| IBIS File
| Lattice Semiconductor Corporation
|[Doc Num]   FPGA-MD-02094  ver. 3.0
[IBIS ver]   4.2
[File name]   ecp5u.ibs
[File Rev]   3.0
[Date]   Mon Mar 10 17:47:18 PDT 2025
[Source]   Lattice Semiconductor umc40lp Process
[Notes]   Device: LFE5U-12F   Final
   Device: LFE5U-25F   Final
   Device: LFE5U-45F   Final
   Device: LFE5U-85F   Final
   Device: LFE5UM-25F   Final
   Device: LFE5UM-45F   Final
   Device: LFE5UM-85F   Final
   Device: LFE5UM5G-25F   Final
   Device: LFE5UM5G-45F   Final
   Device: LFE5UM5G-85F   Final
   Device: LAE5U-12F   Final
   Device: LAE5UM-25F   Final
   Device: LAE5UM-45F   Final
   Device: LAE5UM-85F   Final
   Lattice Semiconductor has worked hard to ensure the
   models below are accurate and complete.  However, the
   data below was generated using simulation of the
   input/output model files for the silicon.  Therefore,
   the data below is for reference and initial design
   purposes only.
   Lattice Semiconductor grants permission to use this
   data for use in printed circuit design using this
   Lattice programmable logic device.  Other use of this
   code, including the selling or duplication of any
   portion is strictly prohibited.
|   NAMING CONVENTION
   The IBIS [Model] header is limited by the specification to a
   total of characters.  With such a set of characters available
   for naming models it becomes important to attempt to
   meaningfully encode the IO standards so they fit within the
   twenty character limit.  It would seem that twenty characters
   would provide room enough for describing IO's.  However, the
   PLD IO structure continues to grow more and more complex.  The
   complexity is making the twenty characters insuffiently
   descriptive.  In order to overcome this issue the naming
   convention described below is implemented to resolve the issue.
The twenty character space is managed as follows:
   bbbvvvsdddprttaaoixx
   b = standard
   v = voltage (x.xx V)
   s = slew code
   d = drive (xx.x ma)
   p = pullmode code
   r = impedance
   t = termination code
   o = diff resistor code
   i = diff  current code
   x = reserved
   standard
   LVCMOS   lvc
   lvcmosd   lvd
   LVDS25e   lve
   LVTTL   lvt
   lvttld   ltd
   sstl_I   ss1
   sstl_II   ss2
   sstld_I   s1d
   sstld_II   s2d
   hsul12   hs1
   hsul12d   h1d
   lvds   lvs
   blvds25   blv
   blvds25e   blv
   mlvds   mlv
   mlvds25e   mle
   lvpecl33   lvp
   lvpecl33e   lvp
   sublvds   slv
   slvs   svs
   slvs15e   sve
   mipi   mip
   vref1   vr1
   slew
   na   a
   fast   f
   slow   s
   pullmode
   off   a
   clamp   e
   impedance
   off   a
   termination
   off   aa
   50   cc
   75   dd
   150   ee
   differential resistor
   off   a
   100   b
   differential current
   NA   a
   3.5   c
   Reserved   IO type
   in   input only
   ou   output
   io   I/O
   od   Open drain
   on   Inverting differential I/O
   (signal name only)
   op   Non-Inverting differential I/O
   (signal name only)
   All the IO models are generated with pull mode set to none.
   Lattice Semiconductor Corporation
   5555 NE Moore Court
   Hillsboro, OR 97214
   U.S.A
   TEL: 1-800-Lattice (USA and Canada)
   408-826-6000 (other locations)
   web: http://www.latticesemi.com/
   email: techsupport@latticesemi.com
The IBIS models by default includes the worst case package data
under [package].  If detailed package model is required , it can be
enable using [package model] keyword.
The .pkg files are included in the zip file with the IBIS models.
The .pkg file has to be located in the same directory as IBIS file.
[Disclaimer] This IBIS source code is intended as a design reference
   which illustrates how the Lattice Semiconductor device operates.
   It is the user's responsibility to verify their design for
   consistency and functionality through the use of formal
   verification methods.  Lattice Semiconductor provides no warranty
   regarding the use or functionality of this data.
[Copyright]   Copyright 2007 by Lattice Semiconductor Corporation
|   Component SAPPHIRE
[Component]   SAPPHIRE
[Manufacturer]   Lattice Semiconductor Corp.
[Package]
|csfBGA285
| variable   typ   min   max
R_pkg   64.450m   23.9m   84m
L_pkg   1.395nH   0.37nH   2.15nH
C_pkg   0.56pF   0.19pF   0.65pF
|caBGA256
| variable   typ   min   max
|R_pkg   301.88m   168.88m   475.12m
|L_pkg   4.862nH   2.153nH   8.583nH
|C_pkg   0.654pF   0.3926pF   1.017pF
|caBGA381
| variable   typ   min   max
|R_pkg   84.450m   81.900m   87.000m
|L_pkg   5.395nH   4.379nH   6.81nH
|C_pkg   0.806pF   0.677pF   1.135pF
|caBGA554
| variable   typ   min   max
|R_pkg   740m   471.54m   505m
|L_pkg   6.1nH   4.8nH   8.1nH
|C_pkg   1.01pF   0.74pF   1.304pF
|caBGA756
| variable   typ   min   max
|R_pkg   284.450m   181.900m   387.000m
|L_pkg   6.395nH   5.379nH   8.411nH
|C_pkg   0.806pF   0.677pF   1.135pF
|caBGA225
| variable   typ   min   max
|R_pkg   219.18m   67.234m   502.9m
|L_pkg   1.301nH   0.5017nH   2.898nH
|C_pkg   0.5201pF   0.3141pF   0.812pF
|TQFP144
| variable   typ   min   max
|R_pkg   0.57206   0.48228   0.73831
|L_pkg   7.596e-9   6.661e-9   8.771e-9
|C_pkg   5.076e-13   4.246e-13   6.163e-13
[Pin]  signal_name   model_name   R_pin   L_pin   C_pin
1   blv250f160eaaaaaaaio   blv250f160eaaaaaaaio
2   blv250s160eaaaaaaaio   blv250s160eaaaaaaaio
3   hs1120f040eaaaaaaaio   hs1120f040eaaaaaaaio
4   hs1120f080eaaaaaaaio   hs1120f080eaaaaaaaio
5   hs1120s040eaaaaaaaio   hs1120s040eaaaaaaaio
6   hs1120s080eaaaaaaaio   hs1120s080eaaaaaaaio
7   lvc120f040eaaaaaaaio   lvc120f040eaaaaaaaio
8   lvc120f080eaaaaaaaio   lvc120f080eaaaaaaaio
9   lvc120s040eaaaaaaaio   lvc120s040eaaaaaaaio
10   lvc120s080eaaaaaaaio   lvc120s080eaaaaaaaio
11   lvc150f040eaaaaaaaio   lvc150f040eaaaaaaaio
12   lvc150f080eaaaaaaaio   lvc150f080eaaaaaaaio
13   lvc150f120eaaaaaaaio   lvc150f120eaaaaaaaio
14   lvc150s040eaaaaaaaio   lvc150s040eaaaaaaaio
15   lvc150s080eaaaaaaaio   lvc150s080eaaaaaaaio
16   lvc150s120eaaaaaaaio   lvc150s120eaaaaaaaio
17   lvc180f040eaaaaaaaio   lvc180f040eaaaaaaaio
18   lvc180f080eaaaaaaaio   lvc180f080eaaaaaaaio
19   lvc180f120eaaaaaaaio   lvc180f120eaaaaaaaio
20   lvc180s040eaaaaaaaio   lvc180s040eaaaaaaaio
21   lvc180s080eaaaaaaaio   lvc180s080eaaaaaaaio
22   lvc180s120eaaaaaaaio   lvc180s120eaaaaaaaio
23   lvc250f040eaaaaaaaio   lvc250f040eaaaaaaaio
24   lvc250f080eaaaaaaaio   lvc250f080eaaaaaaaio
25   lvc250f120eaaaaaaaio   lvc250f120eaaaaaaaio
26   lvc250s040eaaaaaaaio   lvc250s040eaaaaaaaio
27   lvc250s080eaaaaaaaio   lvc250s080eaaaaaaaio
28   lvc250s120eaaaaaaaio   lvc250s120eaaaaaaaio
29   lvc330f040eaaaaaaaio   lvc330f040eaaaaaaaio
30   lvc330f080eaaaaaaaio   lvc330f080eaaaaaaaio
31   lvc330f120eaaaaaaaio   lvc330f120eaaaaaaaio
32   lvc330f160eaaaaaaaio   lvc330f160eaaaaaaaio
33   lvc330s040eaaaaaaaio   lvc330s040eaaaaaaaio
34   lvc330s080eaaaaaaaio   lvc330s080eaaaaaaaio
35   lvc330s120eaaaaaaaio   lvc330s120eaaaaaaaio
36   lvc330s160eaaaaaaaio   lvc330s160eaaaaaaaio
37   mle250f160eaaaaaaaio   mle250f160eaaaaaaaio
38   mle250s160eaaaaaaaio   mle250s160eaaaaaaaio
39   ss1135f080eaaaaaaaio   ss1135f080eaaaaaaaio
40   ss1135s080eaaaaaaaio   ss1135s080eaaaaaaaio
41   ss1150f080eaaaaaaaio   ss1150f080eaaaaaaaio
42   ss1150s080eaaaaaaaio   ss1150s080eaaaaaaaio
43   ss1180f080eaaaaaaaio   ss1180f080eaaaaaaaio
44   ss1180s080eaaaaaaaio   ss1180s080eaaaaaaaio
45   ss2135f100eaaaaaaaio   ss2135f100eaaaaaaaio
46   ss2135s100eaaaaaaaio   ss2135s100eaaaaaaaio
47   ss2150f100eaaaaaaaio   ss2150f100eaaaaaaaio
48   ss2150s100eaaaaaaaio   ss2150s100eaaaaaaaio
49   ss2180f160eaaaaaaaio   ss2180f160eaaaaaaaio
50   ss2180s160eaaaaaaaio   ss2180s160eaaaaaaaio
51   h1d120f080eaaaaaaaio   h1d120f080eaaaaaaaio
52   h1d120s080eaaaaaaaio   h1d120s080eaaaaaaaio
53   h1d120f040eaaaaaaaio   h1d120f040eaaaaaaaio
54   h1d120s040eaaaaaaaio   h1d120s040eaaaaaaaio
55   lvd250f120eaaaaaaaio   lvd250f120eaaaaaaaio
56   lvd250f080eaaaaaaaio   lvd250f080eaaaaaaaio
57   lvd250s080eaaaaaaaio   lvd250s080eaaaaaaaio
58   lvd250s040eaaaaaaaio   lvd250s040eaaaaaaaio
59   lvd250s120eaaaaaaaio   lvd250s120eaaaaaaaio
60   lvd250f040eaaaaaaaio   lvd250f040eaaaaaaaio
61   lvd330f120eaaaaaaaio   lvd330f120eaaaaaaaio
62   lvd330s160eaaaaaaaio   lvd330s160eaaaaaaaio
63   lvd330s040eaaaaaaaio   lvd330s040eaaaaaaaio
64   lvd330f080eaaaaaaaio   lvd330f080eaaaaaaaio
65   lvd330s120eaaaaaaaio   lvd330s120eaaaaaaaio
66   lvd330s080eaaaaaaaio   lvd330s080eaaaaaaaio
67   lvd330f160eaaaaaaaio   lvd330f160eaaaaaaaio
68   lvd330f040eaaaaaaaio   lvd330f040eaaaaaaaio
69   ltd330f120eaaaaaaaio   ltd330f120eaaaaaaaio
70   ltd330s160eaaaaaaaio   ltd330s160eaaaaaaaio
71   ltd330s040eaaaaaaaio   ltd330s040eaaaaaaaio
72   ltd330f080eaaaaaaaio   ltd330f080eaaaaaaaio
73   ltd330s120eaaaaaaaio   ltd330s120eaaaaaaaio
74   ltd330s080eaaaaaaaio   ltd330s080eaaaaaaaio
75   ltd330f160eaaaaaaaio   ltd330f160eaaaaaaaio
76   ltd330f040eaaaaaaaio   ltd330f040eaaaaaaaio
77   lvt330f120eaaaaaaaio   lvt330f120eaaaaaaaio
78   lvt330s160eaaaaaaaio   lvt330s160eaaaaaaaio
79   lvt330s040eaaaaaaaio   lvt330s040eaaaaaaaio
80   lvt330f080eaaaaaaaio   lvt330f080eaaaaaaaio
81   lvt330s120eaaaaaaaio   lvt330s120eaaaaaaaio
82   lvt330s080eaaaaaaaio   lvt330s080eaaaaaaaio
83   lvt330f160eaaaaaaaio   lvt330f160eaaaaaaaio
84   lvt330f040eaaaaaaaio   lvt330f040eaaaaaaaio
85   s1d150s080eaaaaaaaio   s1d150s080eaaaaaaaio
86   s1d150f080eaaaaaaaio   s1d150f080eaaaaaaaio
87   s2d150f100eaaaaaaaio   s2d150f100eaaaaaaaio
88   s2d135s100eaaaaaaaio   s2d135s100eaaaaaaaio
89   s2d150s100eaaaaaaaio   s2d150s100eaaaaaaaio
90   s2d135f100eaaaaaaaio   s2d135f100eaaaaaaaio
91   s2d180f160eaaaaaaaio   s2d180f160eaaaaaaaio
92   s1d135s080eaaaaaaaio   s1d135s080eaaaaaaaio
93   s1d180f080eaaaaaaaio   s1d180f080eaaaaaaaio
94   s2d180s160eaaaaaaaio   s2d180s160eaaaaaaaio
95   s1d135f080eaaaaaaaio   s1d135f080eaaaaaaaio
96   s1d180s080eaaaaaaaio   s1d180s080eaaaaaaaio
97   lvd250f120eaaaaaaaop   lvd250f120eaaaaaaaou
98   lvd250f120eaaaaaaaon   lvd250f120eaaaaaaaou
99   lvc150s040eaaaaaaaou   lvc150s040eaaaaaaaou
100  lvc180f120eaaaaaaaou   lvc180f120eaaaaaaaou
101  ltd330s160eaaaaaaaop   ltd330s160eaaaaaaaou
102  ltd330s160eaaaaaaaon   ltd330s160eaaaaaaaou
103  ss1150f080eaaaaaaaou   ss1150f080eaaaaaaaou
104  s2d150f100eaaaaaaaop   s2d150f100eaaaaaaaou
105  s2d150f100eaaaaaaaon   s2d150f100eaaaaaaaou
106  lvd330s120eaaaaaaaop   lvd330s120eaaaaaaaou
107  lvd330s120eaaaaaaaon   lvd330s120eaaaaaaaou
108  lvc330f080eaaaaaaaou   lvc330f080eaaaaaaaou
109  lvd250f080eaaaaaaaop   lvd250f080eaaaaaaaou
110  lvd250f080eaaaaaaaon   lvd250f080eaaaaaaaou
111  lvc180s120eaaaaaaaou   lvc180s120eaaaaaaaou
112  s2d135f100eaaaaaaaop   s2d135f100eaaaaaaaou
113  s2d135f100eaaaaaaaon   s2d135f100eaaaaaaaou
114  s1d180s080eaaaaaaaop   s1d180s080eaaaaaaaou
115  s1d180s080eaaaaaaaon   s1d180s080eaaaaaaaou
116  lvc180s080eaaaaaaaou   lvc180s080eaaaaaaaou
117  lvc250f120eaaaaaaaou   lvc250f120eaaaaaaaou
118  lvd250s120eaaaaaaaop   lvd250s120eaaaaaaaou
119  lvd250s120eaaaaaaaon   lvd250s120eaaaaaaaou
120  lvc330f040eaaaaaaaou   lvc330f040eaaaaaaaou
121  lvc180f080eaaaaaaaou   lvc180f080eaaaaaaaou
122  ss1150s080eaaaaaaaou   ss1150s080eaaaaaaaou
123  lvc330f120eaaaaaaaou   lvc330f120eaaaaaaaou
124  ss2135s100eaaaaaaaou   ss2135s100eaaaaaaaou
125  lvc120s080eaaaaaaaou   lvc120s080eaaaaaaaou
126  ss2150s100eaaaaaaaou   ss2150s100eaaaaaaaou
127  ss2135f100eaaaaaaaou   ss2135f100eaaaaaaaou
128  s2d180s160eaaaaaaaop   s2d180s160eaaaaaaaou
129  s2d180s160eaaaaaaaon   s2d180s160eaaaaaaaou
130  lvc330s120eaaaaaaaou   lvc330s120eaaaaaaaou
131  h1d120s080eaaaaaaaop   h1d120s080eaaaaaaaou
132  h1d120s080eaaaaaaaon   h1d120s080eaaaaaaaou
133  ss2180f160eaaaaaaaou   ss2180f160eaaaaaaaou
134  lvc330f160eaaaaaaaou   lvc330f160eaaaaaaaou
135  lvd330f080eaaaaaaaop   lvd330f080eaaaaaaaou
136  lvd330f080eaaaaaaaon   lvd330f080eaaaaaaaou
137  s1d180f080eaaaaaaaop   s1d180f080eaaaaaaaou
138  s1d180f080eaaaaaaaon   s1d180f080eaaaaaaaou
139  lvd330s080eaaaaaaaop   lvd330s080eaaaaaaaou
140  lvd330s080eaaaaaaaon   lvd330s080eaaaaaaaou
141  mle250s160eaaaaaaaop   mle250s160eaaaaaaaou
142  mle250s160eaaaaaaaon   mle250s160eaaaaaaaou
143  lvc330s160eaaaaaaaou   lvc330s160eaaaaaaaou
144  lvc180s040eaaaaaaaou   lvc180s040eaaaaaaaou
145  lvc330s040eaaaaaaaou   lvc330s040eaaaaaaaou
146  lvc250s120eaaaaaaaou   lvc250s120eaaaaaaaou
147  lvc250f040eaaaaaaaou   lvc250f040eaaaaaaaou
148  hs1120f080eaaaaaaaou   hs1120f080eaaaaaaaou
149  h1d120f040eaaaaaaaop   h1d120f040eaaaaaaaou
150  h1d120f040eaaaaaaaon   h1d120f040eaaaaaaaou
151  ss1180f080eaaaaaaaou   ss1180f080eaaaaaaaou
152  mle250f160eaaaaaaaop   mle250f160eaaaaaaaou
153  mle250f160eaaaaaaaon   mle250f160eaaaaaaaou
154  lvd250s040eaaaaaaaop   lvd250s040eaaaaaaaou
155  lvd250s040eaaaaaaaon   lvd250s040eaaaaaaaou
156  ltd330f080eaaaaaaaop   ltd330f080eaaaaaaaou
157  ltd330f080eaaaaaaaon   ltd330f080eaaaaaaaou
158  lvd250f040eaaaaaaaop   lvd250f040eaaaaaaaou
159  lvd250f040eaaaaaaaon   lvd250f040eaaaaaaaou
160  lvc150f080eaaaaaaaou   lvc150f080eaaaaaaaou
161  lvc330s080eaaaaaaaou   lvc330s080eaaaaaaaou
162  lvc120s040eaaaaaaaou   lvc120s040eaaaaaaaou
163  s2d180f160eaaaaaaaop   s2d180f160eaaaaaaaou
164  s2d180f160eaaaaaaaon   s2d180f160eaaaaaaaou
165  ss1135f080eaaaaaaaou   ss1135f080eaaaaaaaou
166  ltd330s120eaaaaaaaop   ltd330s120eaaaaaaaou
167  ltd330s120eaaaaaaaon   ltd330s120eaaaaaaaou
168  lvc120f040eaaaaaaaou   lvc120f040eaaaaaaaou
169  lvc150s080eaaaaaaaou   lvc150s080eaaaaaaaou
170  lvc250s080eaaaaaaaou   lvc250s080eaaaaaaaou
171  s2d135s100eaaaaaaaop   s2d135s100eaaaaaaaou
172  s2d135s100eaaaaaaaon   s2d135s100eaaaaaaaou
173  ltd330f160eaaaaaaaop   ltd330f160eaaaaaaaou
174  ltd330f160eaaaaaaaon   ltd330f160eaaaaaaaou
175  lvc250s040eaaaaaaaou   lvc250s040eaaaaaaaou
176  lvd330s160eaaaaaaaop   lvd330s160eaaaaaaaou
177  lvd330s160eaaaaaaaon   lvd330s160eaaaaaaaou
178  s1d135s080eaaaaaaaop   s1d135s080eaaaaaaaou
179  s1d135s080eaaaaaaaon   s1d135s080eaaaaaaaou
180  lvc180f040eaaaaaaaou   lvc180f040eaaaaaaaou
181  lvc120f080eaaaaaaaou   lvc120f080eaaaaaaaou
182  blv250s160eaaaaaaaop   blv250s160eaaaaaaaou
183  blv250s160eaaaaaaaon   blv250s160eaaaaaaaou
184  ltd330s080eaaaaaaaop   ltd330s080eaaaaaaaou
185  ltd330s080eaaaaaaaon   ltd330s080eaaaaaaaou
186  h1d120s040eaaaaaaaop   h1d120s040eaaaaaaaou
187  h1d120s040eaaaaaaaon   h1d120s040eaaaaaaaou
188  lvd250s080eaaaaaaaop   lvd250s080eaaaaaaaou
189  lvd250s080eaaaaaaaon   lvd250s080eaaaaaaaou
190  lvd330f040eaaaaaaaop   lvd330f040eaaaaaaaou
191  lvd330f040eaaaaaaaon   lvd330f040eaaaaaaaou
192  ss1135s080eaaaaaaaou   ss1135s080eaaaaaaaou
193  ss2180s160eaaaaaaaou   ss2180s160eaaaaaaaou
194  hs1120f040eaaaaaaaou   hs1120f040eaaaaaaaou
195  hs1120s040eaaaaaaaou   hs1120s040eaaaaaaaou
196  s1d150f080eaaaaaaaop   s1d150f080eaaaaaaaou
197  s1d150f080eaaaaaaaon   s1d150f080eaaaaaaaou
198  ltd330s040eaaaaaaaop   ltd330s040eaaaaaaaou
199  ltd330s040eaaaaaaaon   ltd330s040eaaaaaaaou
200  ltd330f120eaaaaaaaop   ltd330f120eaaaaaaaou
201  ltd330f120eaaaaaaaon   ltd330f120eaaaaaaaou
202  lvc250f080eaaaaaaaou   lvc250f080eaaaaaaaou
203  s2d150s100eaaaaaaaop   s2d150s100eaaaaaaaou
204  s2d150s100eaaaaaaaon   s2d150s100eaaaaaaaou
205  ltd330f040eaaaaaaaop   ltd330f040eaaaaaaaou
206  ltd330f040eaaaaaaaon   ltd330f040eaaaaaaaou
207  s1d150s080eaaaaaaaop   s1d150s080eaaaaaaaou
208  s1d150s080eaaaaaaaon   s1d150s080eaaaaaaaou
209  blv250f160eaaaaaaaop   blv250f160eaaaaaaaou
210  blv250f160eaaaaaaaon   blv250f160eaaaaaaaou
211  lvd330f120eaaaaaaaop   lvd330f120eaaaaaaaou
212  lvd330f120eaaaaaaaon   lvd330f120eaaaaaaaou
213  h1d120f080eaaaaaaaop   h1d120f080eaaaaaaaou
214  h1d120f080eaaaaaaaon   h1d120f080eaaaaaaaou
215  lvd330s040eaaaaaaaop   lvd330s040eaaaaaaaou
216  lvd330s040eaaaaaaaon   lvd330s040eaaaaaaaou
217  lvd330f160eaaaaaaaop   lvd330f160eaaaaaaaou
218  lvd330f160eaaaaaaaon   lvd330f160eaaaaaaaou
219  ss2150f100eaaaaaaaou   ss2150f100eaaaaaaaou
220  s1d135f080eaaaaaaaop   s1d135f080eaaaaaaaou
221  s1d135f080eaaaaaaaon   s1d135f080eaaaaaaaou
222  hs1120s080eaaaaaaaou   hs1120s080eaaaaaaaou
223  lvc150f040eaaaaaaaou   lvc150f040eaaaaaaaou
224  ss1180s080eaaaaaaaou   ss1180s080eaaaaaaaou
225  ss1150s080eaccaaaaio   ss1150s080eaccaaaaio
226  ss1150f080eaccaaaaio   ss1150f080eaccaaaaio
227  ss2150f100eaccaaaaio   ss2150f100eaccaaaaio
228  ss2135s100eaccaaaaio   ss2135s100eaccaaaaio
229  ss2150s100eaccaaaaio   ss2150s100eaccaaaaio
230  ss2135f100eaccaaaaio   ss2135f100eaccaaaaio
231  ss2180f160eaccaaaaio   ss2180f160eaccaaaaio
232  ss1135s080eaccaaaaio   ss1135s080eaccaaaaio
233  ss1180f080eaccaaaaio   ss1180f080eaccaaaaio
234  ss2180s160eaccaaaaio   ss2180s160eaccaaaaio
235  ss1135f080eaccaaaaio   ss1135f080eaccaaaaio
236  ss1180s080eaccaaaaio   ss1180s080eaccaaaaio
237  ss1150s080eaddaaaaio   ss1150s080eaddaaaaio
238  ss1150f080eaddaaaaio   ss1150f080eaddaaaaio
239  ss2150f100eaddaaaaio   ss2150f100eaddaaaaio
240  ss2135s100eaddaaaaio   ss2135s100eaddaaaaio
241  ss2150s100eaddaaaaio   ss2150s100eaddaaaaio
242  ss2135f100eaddaaaaio   ss2135f100eaddaaaaio
243  ss2180f160eaddaaaaio   ss2180f160eaddaaaaio
244  ss1135s080eaddaaaaio   ss1135s080eaddaaaaio
245  ss1180f080eaddaaaaio   ss1180f080eaddaaaaio
246  ss2180s160eaddaaaaio   ss2180s160eaddaaaaio
247  ss1135f080eaddaaaaio   ss1135f080eaddaaaaio
248  ss1180s080eaddaaaaio   ss1180s080eaddaaaaio
249  ss1150s080eaeeaaaaio   ss1150s080eaeeaaaaio
250  ss1150f080eaeeaaaaio   ss1150f080eaeeaaaaio
251  ss2150f100eaeeaaaaio   ss2150f100eaeeaaaaio
252  ss2135s100eaeeaaaaio   ss2135s100eaeeaaaaio
253  ss2150s100eaeeaaaaio   ss2150s100eaeeaaaaio
254  ss2135f100eaeeaaaaio   ss2135f100eaeeaaaaio
255  ss2180f160eaeeaaaaio   ss2180f160eaeeaaaaio
256  ss1135s080eaeeaaaaio   ss1135s080eaeeaaaaio
257  ss1180f080eaeeaaaaio   ss1180f080eaeeaaaaio
258  ss2180s160eaeeaaaaio   ss2180s160eaeeaaaaio
259  ss1135f080eaeeaaaaio   ss1135f080eaeeaaaaio
260  ss1180s080eaeeaaaaio   ss1180s080eaeeaaaaio
261  s1d150s080eaaaaabaio   s1d150s080eaaaaabaio
262  s1d150f080eaaaaabaio   s1d150f080eaaaaabaio
263  s2d150f100eaaaaabaio   s2d150f100eaaaaabaio
264  s2d135s100eaaaaabaio   s2d135s100eaaaaabaio
265  s2d150s100eaaaaabaio   s2d150s100eaaaaabaio
266  s2d135f100eaaaaabaio   s2d135f100eaaaaabaio
267  s2d180f160eaaaaabaio   s2d180f160eaaaaabaio
268  s1d135s080eaaaaabaio   s1d135s080eaaaaabaio
269  s1d180f080eaaaaabaio   s1d180f080eaaaaabaio
270  s2d180s160eaaaaabaio   s2d180s160eaaaaabaio
271  s1d135f080eaaaaabaio   s1d135f080eaaaaabaio
272  lvt330s120eaaaaaaaou   lvt330s120eaaaaaaaou
273  lvt330f080eaaaaaaaou   lvt330f080eaaaaaaaou
274  lvt330s080eaaaaaaaou   lvt330s080eaaaaaaaou
275  lvt330s160eaaaaaaaou   lvt330s160eaaaaaaaou
276  lvt330s040eaaaaaaaou   lvt330s040eaaaaaaaou
277  lvt330f160eaaaaaaaou   lvt330f160eaaaaaaaou
278  lve250f080eaaaaaaaou   lve250f080eaaaaaaaou
279  s1d180s080eaaaaabaio   s1d180s080eaaaaabaio
280  lvt330f120eaaaaaaaou   lvt330f120eaaaaaaaou
281  lvt330f040eaaaaaaaou   lvt330f040eaaaaaaaou
282  lve250s080eaaaaaaaou   lve250s080eaaaaaaaou
283  lvp330s160eaaaaaaaop   lvp330s160eaaaaaaaou
284  lvp330s160eaaaaaaaon   lvp330s160eaaaaaaaou
285  lvp330f160eaaaaaaaop   lvp330f160eaaaaaaaou
286  lvp330f160eaaaaaaaon   lvp330f160eaaaaaaaou
287  lvc150s040eaaaaaaaod   lvc150s040eaaaaaaaod
288  lvc180f120eaaaaaaaod   lvc180f120eaaaaaaaod
289  lvt330s160eaaaaaaaod   lvt330s160eaaaaaaaod
290  lvc330f080eaaaaaaaod   lvc330f080eaaaaaaaod
291  lvc180s120eaaaaaaaod   lvc180s120eaaaaaaaod
292  lvc180s080eaaaaaaaod   lvc180s080eaaaaaaaod
293  lvc250f120eaaaaaaaod   lvc250f120eaaaaaaaod
294  lvt330s120eaaaaaaaod   lvt330s120eaaaaaaaod
295  lvc330f040eaaaaaaaod   lvc330f040eaaaaaaaod
296  lvc180f080eaaaaaaaod   lvc180f080eaaaaaaaod
297  lvc330f120eaaaaaaaod   lvc330f120eaaaaaaaod
298  lvc120s080eaaaaaaaod   lvc120s080eaaaaaaaod
299  lvc330s120eaaaaaaaod   lvc330s120eaaaaaaaod
300  lvc330f160eaaaaaaaod   lvc330f160eaaaaaaaod
301  lvc330s160eaaaaaaaod   lvc330s160eaaaaaaaod
302  lvc180s040eaaaaaaaod   lvc180s040eaaaaaaaod
303  lvc330s040eaaaaaaaod   lvc330s040eaaaaaaaod
304  lvc250s120eaaaaaaaod   lvc250s120eaaaaaaaod
305  lvc250f040eaaaaaaaod   lvc250f040eaaaaaaaod
306  lvc150f080eaaaaaaaod   lvc150f080eaaaaaaaod
307  lvc330s080eaaaaaaaod   lvc330s080eaaaaaaaod
308  lvc120s040eaaaaaaaod   lvc120s040eaaaaaaaod
309  lvt330f120eaaaaaaaod   lvt330f120eaaaaaaaod
310  lvc120f040eaaaaaaaod   lvc120f040eaaaaaaaod
311  lvc150s080eaaaaaaaod   lvc150s080eaaaaaaaod
312  lvc250s080eaaaaaaaod   lvc250s080eaaaaaaaod
313  lvc250s040eaaaaaaaod   lvc250s040eaaaaaaaod
314  lvt330s040eaaaaaaaod   lvt330s040eaaaaaaaod
315  lvc180f040eaaaaaaaod   lvc180f040eaaaaaaaod
316  lvt330f160eaaaaaaaod   lvt330f160eaaaaaaaod
317  lvc120f080eaaaaaaaod   lvc120f080eaaaaaaaod
318  lvt330f080eaaaaaaaod   lvt330f080eaaaaaaaod
319  lvt330s080eaaaaaaaod   lvt330s080eaaaaaaaod
320  lvc250f080eaaaaaaaod   lvc250f080eaaaaaaaod
321  lvt330f040eaaaaaaaod   lvt330f040eaaaaaaaod
322  lvc150f040eaaaaaaaod   lvc150f040eaaaaaaaod
323  lvc150s040aaaaaaaaod   lvc150s040aaaaaaaaod
324  lvc180f120aaaaaaaaod   lvc180f120aaaaaaaaod
325  lvt330s160aaaaaaaaod   lvt330s160aaaaaaaaod
326  lvc330f080aaaaaaaaod   lvc330f080aaaaaaaaod
327  lvc180s120aaaaaaaaod   lvc180s120aaaaaaaaod
328  lvc180s080aaaaaaaaod   lvc180s080aaaaaaaaod
329  lvc250f120aaaaaaaaod   lvc250f120aaaaaaaaod
330  lvt330s120aaaaaaaaod   lvt330s120aaaaaaaaod
331  lvc330f040aaaaaaaaod   lvc330f040aaaaaaaaod
332  lvc180f080aaaaaaaaod   lvc180f080aaaaaaaaod
333  lvc330f120aaaaaaaaod   lvc330f120aaaaaaaaod
334  lvc120s080aaaaaaaaod   lvc120s080aaaaaaaaod
335  lvc330s120aaaaaaaaod   lvc330s120aaaaaaaaod
336  lvc330f160aaaaaaaaod   lvc330f160aaaaaaaaod
337  lvc330s160aaaaaaaaod   lvc330s160aaaaaaaaod
338  lvc180s040aaaaaaaaod   lvc180s040aaaaaaaaod
339  lvc330s040aaaaaaaaod   lvc330s040aaaaaaaaod
340  lvc250s120aaaaaaaaod   lvc250s120aaaaaaaaod
341  lvc250f040aaaaaaaaod   lvc250f040aaaaaaaaod
342  lvc150f080aaaaaaaaod   lvc150f080aaaaaaaaod
343  lvc330s080aaaaaaaaod   lvc330s080aaaaaaaaod
344  lvc120s040aaaaaaaaod   lvc120s040aaaaaaaaod
345  lvt330f120aaaaaaaaod   lvt330f120aaaaaaaaod
346  lvc120f040aaaaaaaaod   lvc120f040aaaaaaaaod
347  lvc150s080aaaaaaaaod   lvc150s080aaaaaaaaod
348  lvc250s080aaaaaaaaod   lvc250s080aaaaaaaaod
349  lvc250s040aaaaaaaaod   lvc250s040aaaaaaaaod
350  lvt330s040aaaaaaaaod   lvt330s040aaaaaaaaod
351  lvc180f040aaaaaaaaod   lvc180f040aaaaaaaaod
352  lvt330f160aaaaaaaaod   lvt330f160aaaaaaaaod
353  lvc120f080aaaaaaaaod   lvc120f080aaaaaaaaod
354  lvt330f080aaaaaaaaod   lvt330f080aaaaaaaaod
355  lvt330s080aaaaaaaaod   lvt330s080aaaaaaaaod
356  lvc250f080aaaaaaaaod   lvc250f080aaaaaaaaod
357  lvt330f040aaaaaaaaod   lvt330f040aaaaaaaaod
358  lvc150f040aaaaaaaaod   lvc150f040aaaaaaaaod
359  lvc120f120aaaaaaaaod   lvc120f120aaaaaaaaod
360  lvc120s120aaaaaaaaod   lvc120s120aaaaaaaaod
361  lvc150f120aaaaaaaaod   lvc150f120aaaaaaaaod
362  lvc150s120aaaaaaaaod   lvc150s120aaaaaaaaod
363  lvc180f160aaaaaaaaod   lvc180f160aaaaaaaaod
364  lvc180s160aaaaaaaaod   lvc180s160aaaaaaaaod
365  lvc250f160aaaaaaaaod   lvc250f160aaaaaaaaod
366  lvc250s160aaaaaaaaod   lvc250s160aaaaaaaaod
367  lvc120f120eaaaaaaaod   lvc120f120eaaaaaaaod
368  lvc120s120eaaaaaaaod   lvc120s120eaaaaaaaod
369  lvc150f120eaaaaaaaod   lvc150f120eaaaaaaaod
370  lvc150s120eaaaaaaaod   lvc150s120eaaaaaaaod
371  lvc180f160eaaaaaaaod   lvc180f160eaaaaaaaod
372  lvc180s160eaaaaaaaod   lvc180s160eaaaaaaaod
373  lvc250f160eaaaaaaaod   lvc250f160eaaaaaaaod
374  lvc250s160eaaaaaaaod   lvc250s160eaaaaaaaod
375  lvc120f160aaaaaaaaod   lvc120f160aaaaaaaaod
376  lvc120f160eaaaaaaaod   lvc120f160eaaaaaaaod
377  lvc120s160aaaaaaaaod   lvc120s160aaaaaaaaod
378  lvc120s160eaaaaaaaod   lvc120s160eaaaaaaaod
379  lvc150f160aaaaaaaaod   lvc150f160aaaaaaaaod
380  lvc150f160eaaaaaaaod   lvc150f160eaaaaaaaod
381  lvc150s160aaaaaaaaod   lvc150s160aaaaaaaaod
382  lvc150s160eaaaaaaaod   lvc150s160eaaaaaaaod
383  lvs250axxxeaaaaaacio   lvs250axxxeaaaaaacio
384  lvs250axxxeaaaaaacop   lvs250axxxeaaaaaacou
385  lvs250axxxeaaaaaacon   lvs250axxxeaaaaaacou
386  blv250axxxeaaaaaaain   blv250axxxeaaaaaaain
387  h1d120axxxeaaaaaaain   h1d120axxxeaaaaaaain
388  hs1120axxxeaaaaaaain   hs1120axxxeaaaaaaain
389  ltd330axxxeaaaaaaain   ltd330axxxeaaaaaaain
390  lvc120axxxeaaaaaaain   lvc120axxxeaaaaaaain
391  lvc150axxxeaaaaaaain   lvc150axxxeaaaaaaain
392  lvc180axxxeaaaaaaain   lvc180axxxeaaaaaaain
393  lvc250axxxaaaaaaaain   lvc250axxxaaaaaaaain
394  lvc250axxxeaaaaaaain   lvc250axxxeaaaaaaain
395  lvc330axxxaaaaaaaain   lvc330axxxaaaaaaaain
396  lvc330axxxeaaaaaaain   lvc330axxxeaaaaaaain
397  lvd250axxxeaaaaaaain   lvd250axxxeaaaaaaain
398  lvd330axxxeaaaaaaain   lvd330axxxeaaaaaaain
399  lvp330axxxeaaaaaaain   lvp330axxxeaaaaaaain
400  lvs250axxxeaaaaaaain   lvs250axxxeaaaaaaain
401  lvt330axxxaaaaaaaain   lvt330axxxaaaaaaaain
402  lvt330axxxeaaaaaaain   lvt330axxxeaaaaaaain
403  mlv250axxxeaaaaaaain   mlv250axxxeaaaaaaain
404  s1d135axxxeaaaaaaain   s1d135axxxeaaaaaaain
405  s1d150axxxeaaaaaaain   s1d150axxxeaaaaaaain
406  s1d180axxxeaaaaaaain   s1d180axxxeaaaaaaain
407  s2d135axxxeaaaaaaain   s2d135axxxeaaaaaaain
408  s2d150axxxeaaaaaaain   s2d150axxxeaaaaaaain
409  s2d180axxxeaaaaaaain   s2d180axxxeaaaaaaain
410  slv250axxxeaaaaaaain   slv250axxxeaaaaaaain
411  ss1135axxxeaaaaaaain   ss1135axxxeaaaaaaain
412  ss1135axxxeaccaaaain   ss1135axxxeaccaaaain
413  ss1135axxxeaddaaaain   ss1135axxxeaddaaaain
414  ss1135axxxeaeeaaaain   ss1135axxxeaeeaaaain
415  ss1150axxxeaaaaaaain   ss1150axxxeaaaaaaain
416  ss1150axxxeaccaaaain   ss1150axxxeaccaaaain
417  ss1150axxxeaddaaaain   ss1150axxxeaddaaaain
418  ss1150axxxeaeeaaaain   ss1150axxxeaeeaaaain
419  ss1180axxxeaaaaaaain   ss1180axxxeaaaaaaain
420  ss1180axxxeaccaaaain   ss1180axxxeaccaaaain
421  ss1180axxxeaddaaaain   ss1180axxxeaddaaaain
422  ss1180axxxeaeeaaaain   ss1180axxxeaeeaaaain
423  ss2135axxxeaaaaaaain   ss2135axxxeaaaaaaain
424  ss2135axxxeaccaaaain   ss2135axxxeaccaaaain
425  ss2135axxxeaddaaaain   ss2135axxxeaddaaaain
426  ss2135axxxeaeeaaaain   ss2135axxxeaeeaaaain
427  ss2150axxxeaaaaaaain   ss2150axxxeaaaaaaain
428  ss2150axxxeaccaaaain   ss2150axxxeaccaaaain
429  ss2150axxxeaddaaaain   ss2150axxxeaddaaaain
430  ss2150axxxeaeeaaaain   ss2150axxxeaeeaaaain
431  ss2180axxxeaaaaaaain   ss2180axxxeaaaaaaain
432  ss2180axxxeaccaaaain   ss2180axxxeaccaaaain
433  ss2180axxxeaddaaaain   ss2180axxxeaddaaaain
434  ss2180axxxeaeeaaaain   ss2180axxxeaeeaaaain
435  svs120axxxeaaaaaaain   svs120axxxeaaaaaaain
436  s2d180axxxeaaaaabain   s2d180axxxeaaaaabain
437  mip150axxxeaaaaabain   mip150axxxeaaaaabain
438  svs120axxxeaaaaabain   svs120axxxeaaaaabain
439  s1d150axxxeaaaaabain   s1d150axxxeaaaaabain
440  s1d135axxxeaaaaabain   s1d135axxxeaaaaabain
441  s2d135axxxeaaaaabain   s2d135axxxeaaaaabain
442  lvs250axxxeaaaaabain   lvs250axxxeaaaaabain
443  s1d180axxxeaaaaabain   s1d180axxxeaaaaabain
444  slv250axxxeaaaaabain   slv250axxxeaaaaabain
445  mlv250axxxeaaaaabain   mlv250axxxeaaaaabain
446  lvp330axxxeaaaaabain   lvp330axxxeaaaaabain
447  blv250axxxeaaaaabain   blv250axxxeaaaaabain
448  s2d150axxxeaaaaabain   s2d150axxxeaaaaabain
449  s1d150s080eaccaaaaio   s1d150s080eaccaaaaio
450  s1d150f080eaccaaaaio   s1d150f080eaccaaaaio
451  s2d150f100eaccaaaaio   s2d150f100eaccaaaaio
452  s2d135s100eaccaaaaio   s2d135s100eaccaaaaio
453  s2d150s100eaccaaaaio   s2d150s100eaccaaaaio
454  s2d135f100eaccaaaaio   s2d135f100eaccaaaaio
455  s2d180f160eaccaaaaio   s2d180f160eaccaaaaio
456  s1d135s080eaccaaaaio   s1d135s080eaccaaaaio
457  s1d180f080eaccaaaaio   s1d180f080eaccaaaaio
458  s2d180s160eaccaaaaio   s2d180s160eaccaaaaio
459  s1d135f080eaccaaaaio   s1d135f080eaccaaaaio
460  s1d180s080eaccaaaaio   s1d180s080eaccaaaaio
461  s1d150s080eaddaaaaio   s1d150s080eaddaaaaio
462  s1d150f080eaddaaaaio   s1d150f080eaddaaaaio
463  s2d150f100eaddaaaaio   s2d150f100eaddaaaaio
464  s2d135s100eaddaaaaio   s2d135s100eaddaaaaio
465  s2d150s100eaddaaaaio   s2d150s100eaddaaaaio
466  s2d135f100eaddaaaaio   s2d135f100eaddaaaaio
467  s2d180f160eaddaaaaio   s2d180f160eaddaaaaio
468  s1d135s080eaddaaaaio   s1d135s080eaddaaaaio
469  s1d180f080eaddaaaaio   s1d180f080eaddaaaaio
470  s2d180s160eaddaaaaio   s2d180s160eaddaaaaio
471  s1d135f080eaddaaaaio   s1d135f080eaddaaaaio
472  s1d180s080eaddaaaaio   s1d180s080eaddaaaaio
473  s1d150s080eaeeaaaaio   s1d150s080eaeeaaaaio
474  s1d150f080eaeeaaaaio   s1d150f080eaeeaaaaio
475  s2d150f100eaeeaaaaio   s2d150f100eaeeaaaaio
476  s2d135s100eaeeaaaaio   s2d135s100eaeeaaaaio
477  s2d150s100eaeeaaaaio   s2d150s100eaeeaaaaio
478  s2d135f100eaeeaaaaio   s2d135f100eaeeaaaaio
479  s2d180f160eaeeaaaaio   s2d180f160eaeeaaaaio
480  s1d135s080eaeeaaaaio   s1d135s080eaeeaaaaio
481  s1d180f080eaeeaaaaio   s1d180f080eaeeaaaaio
482  s2d180s160eaeeaaaaio   s2d180s160eaeeaaaaio
483  s1d135f080eaeeaaaaio   s1d135f080eaeeaaaaio
484  s1d180s080eaeeaaaaio   s1d180s080eaeeaaaaio
485  GND   GND
486  POWER   POWER
[Diff pin]  inv_pin  vdiff  tdelay_typ  tdelay_min  tdelay_max
97   98   0.1   0.0s   0.0s   0.0s
101   102   0.1   0.0s   0.0s   0.0s
104   105   0.1   0.0s   0.0s   0.0s
106   107   0.1   0.0s   0.0s   0.0s
109   110   0.1   0.0s   0.0s   0.0s
112   113   0.1   0.0s   0.0s   0.0s
114   115   0.1   0.0s   0.0s   0.0s
118   119   0.1   0.0s   0.0s   0.0s
128   129   0.1   0.0s   0.0s   0.0s
131   132   0.1   0.0s   0.0s   0.0s
135   136   0.1   0.0s   0.0s   0.0s
137   138   0.1   0.0s   0.0s   0.0s
139   140   0.1   0.0s   0.0s   0.0s
141   142   0.1   0.0s   0.0s   0.0s
149   150   0.1   0.0s   0.0s   0.0s
152   153   0.1   0.0s   0.0s   0.0s
154   155   0.1   0.0s   0.0s   0.0s
156   157   0.1   0.0s   0.0s   0.0s
158   159   0.1   0.0s   0.0s   0.0s
163   164   0.1   0.0s   0.0s   0.0s
166   167   0.1   0.0s   0.0s   0.0s
171   172   0.1   0.0s   0.0s   0.0s
173   174   0.1   0.0s   0.0s   0.0s
176   177   0.1   0.0s   0.0s   0.0s
178   179   0.1   0.0s   0.0s   0.0s
182   183   0.1   0.0s   0.0s   0.0s
184   185   0.1   0.0s   0.0s   0.0s
186   187   0.1   0.0s   0.0s   0.0s
188   189   0.1   0.0s   0.0s   0.0s
190   191   0.1   0.0s   0.0s   0.0s
196   197   0.1   0.0s   0.0s   0.0s
198   199   0.1   0.0s   0.0s   0.0s
200   201   0.1   0.0s   0.0s   0.0s
203   204   0.1   0.0s   0.0s   0.0s
205   206   0.1   0.0s   0.0s   0.0s
207   208   0.1   0.0s   0.0s   0.0s
209   210   0.1   0.0s   0.0s   0.0s
211   212   0.1   0.0s   0.0s   0.0s
213   214   0.1   0.0s   0.0s   0.0s
215   216   0.1   0.0s   0.0s   0.0s
217   218   0.1   0.0s   0.0s   0.0s
220   221   0.1   0.0s   0.0s   0.0s
283   284   0.1   0.0s   0.0s   0.0s
285   286   0.1   0.0s   0.0s   0.0s
384   385   0.1   0.0s   0.0s   0.0s
| Models and submodels in the file (439): blv250f160eaaaaaaaio (I/O), blv250s160eaaaaaaaio (I/O), hs1120f040eaaaaaaaio (I/O), hs1120f080eaaaaaaaio (I/O), hs1120s040eaaaaaaaio (I/O), hs1120s080eaaaaaaaio (I/O), lvc120f040eaaaaaaaio (I/O), lvc120f080eaaaaaaaio (I/O), lvc120s040eaaaaaaaio (I/O), lvc120s080eaaaaaaaio (I/O), lvc150f040eaaaaaaaio (I/O), lvc150f080eaaaaaaaio (I/O), lvc150f120eaaaaaaaio (I/O), lvc150s040eaaaaaaaio (I/O), lvc150s080eaaaaaaaio (I/O), lvc150s120eaaaaaaaio (I/O), lvc180f040eaaaaaaaio (I/O), lvc180f080eaaaaaaaio (I/O), lvc180f120eaaaaaaaio (I/O), lvc180s040eaaaaaaaio (I/O), lvc180s080eaaaaaaaio (I/O), lvc180s120eaaaaaaaio (I/O), lvc250f040eaaaaaaaio (I/O), lvc250f080eaaaaaaaio (I/O), lvc250f120eaaaaaaaio (I/O), lvc250s040eaaaaaaaio (I/O), lvc250s080eaaaaaaaio (I/O), lvc250s120eaaaaaaaio (I/O), lvc330f040eaaaaaaaio (I/O), lvc330f080eaaaaaaaio (I/O), lvc330f120eaaaaaaaio (I/O), lvc330f160eaaaaaaaio (I/O), lvc330s040eaaaaaaaio (I/O), lvc330s080eaaaaaaaio (I/O), lvc330s120eaaaaaaaio (I/O), lvc330s160eaaaaaaaio (I/O), mle250f160eaaaaaaaio (I/O), mle250s160eaaaaaaaio (I/O), ss1135f080eaaaaaaaio (I/O), ss1135s080eaaaaaaaio (I/O), ss1150f080eaaaaaaaio (I/O), ss1150s080eaaaaaaaio (I/O), ss1180f080eaaaaaaaio (I/O), ss1180s080eaaaaaaaio (I/O), ss2135f100eaaaaaaaio (I/O), ss2135s100eaaaaaaaio (I/O), ss2150f100eaaaaaaaio (I/O), ss2150s100eaaaaaaaio (I/O), ss2180f160eaaaaaaaio (I/O), ss2180s160eaaaaaaaio (I/O), h1d120f080eaaaaaaaio (I/O), h1d120s080eaaaaaaaio (I/O), h1d120f040eaaaaaaaio (I/O), h1d120s040eaaaaaaaio (I/O), lvd250f120eaaaaaaaio (I/O), lvd250f080eaaaaaaaio (I/O), lvd250s080eaaaaaaaio (I/O), lvd250s040eaaaaaaaio (I/O), lvd250s120eaaaaaaaio (I/O), lvd250f040eaaaaaaaio (I/O), lvd330f120eaaaaaaaio (I/O), lvd330s160eaaaaaaaio (I/O), lvd330s040eaaaaaaaio (I/O), lvd330f080eaaaaaaaio (I/O), lvd330s120eaaaaaaaio (I/O), lvd330s080eaaaaaaaio (I/O), lvd330f160eaaaaaaaio (I/O), lvd330f040eaaaaaaaio (I/O), ltd330f120eaaaaaaaio (I/O), ltd330s160eaaaaaaaio (I/O), ltd330s040eaaaaaaaio (I/O), ltd330f080eaaaaaaaio (I/O), ltd330s120eaaaaaaaio (I/O), ltd330s080eaaaaaaaio (I/O), ltd330f160eaaaaaaaio (I/O), ltd330f040eaaaaaaaio (I/O), lvt330f120eaaaaaaaio (I/O), lvt330s160eaaaaaaaio (I/O), lvt330s040eaaaaaaaio (I/O), lvt330f080eaaaaaaaio (I/O)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
